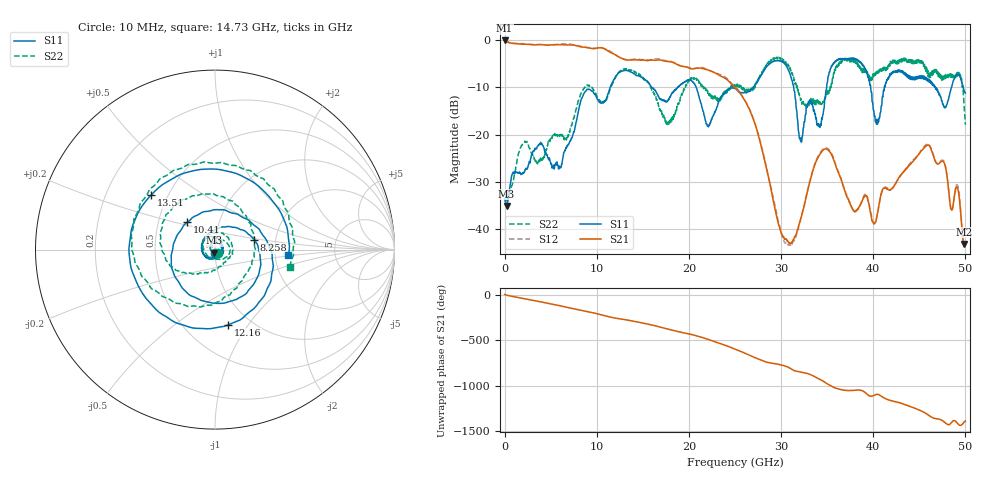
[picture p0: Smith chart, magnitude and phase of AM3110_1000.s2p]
# Hz S DB R 50.0
!freq dBS11 angS11 dBS21 angS21 dBS12 angS12 dBS22 angS22
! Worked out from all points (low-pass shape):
!   1601 points, 10 MHz to 50 GHz, reference 50 ohm
!   highest |S21| = -0.06 dB at 10 MHz (marker M1); lowest = -43.2 dB at 49.88 GHz (marker M2)
!   |S21| within 3 dB of the highest: start of sweep to 11.98 GHz
!   lowest |S11| = -35.2 dB at 228.7 MHz (marker M3), VSWR 1.04, Z = 49.4 - j1.61 ohm
!   |S11| at or under -10 dB: start of sweep to 11.45 GHz; 20.78 GHz to 26.98 GHz (6.198 GHz wide, 26 % of centre); 31.37 GHz to 34.95 GHz (3.575 GHz wide, 10.8 % of centre)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
!   |S22| runs from -34.1 to -3.6 dB; largest |S21 - S12| = 0.027
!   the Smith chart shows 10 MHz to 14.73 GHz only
!   S11 on the Smith chart (normalised r, x): 10 MHz: 1.00, -0.04; 8.258 GHz: 1.55, +0.18; 10.41 GHz: 0.70, +0.22; 12.16 GHz: 0.79, -0.81; 13.51 GHz: 0.40, +0.32; 14.73 GHz: 2.37, -0.18
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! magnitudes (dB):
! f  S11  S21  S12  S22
! 10 MHz  -33.6  -0.1  -0.1  -32.2
! 228.7 MHz  -35.2  -0.3  -0.2  -33.9
! 3.79 GHz  -22.0  -0.9  -0.9  -25.3
! 6.04 GHz  -26.9  -0.9  -0.8  -20.0
! 8.258 GHz  -13.0  -1.4  -1.3  -11.5
! 8.352 GHz  -12.4  -1.4  -1.3  -11.1
! 10.41 GHz  -13.3  -1.6  -1.7  -12.9
! 12.16 GHz  -7.4  -3.3  -3.3  -7.5
! 13.51 GHz  -6.6  -4.2  -4.1  -6.3
! 14.73 GHz  -7.8  -4.2  -4.1  -7.3
! 16.69 GHz  -11.9  -4.2  -3.9  -13.8
! 25 GHz  -10.3  -10.1  -9.9  -9.6
! 30.54 GHz  -5.4  -42.2  -42.9  -4.8
! 32.1 GHz  -21.2  -38.2  -38.2  -12.2
! 33.35 GHz  -13.2  -28.4  -28.2  -12.7
! 35.1 GHz  -7.8  -23.3  -23.0  -10.6
! 38 GHz  -3.8  -36.4  -36.4  -4.3
! 40.47 GHz  -17.8  -36.7  -36.5  -6.9
! 41.69 GHz  -7.8  -31.7  -31.5  -5.9
! 46 GHz  -8.3  -22.2  -22.0  -7.0
! 49.88 GHz  -10.7  -43.2  -43.2  -14.5
! 50 GHz  -11.2  -43.0  -42.8  -17.9
